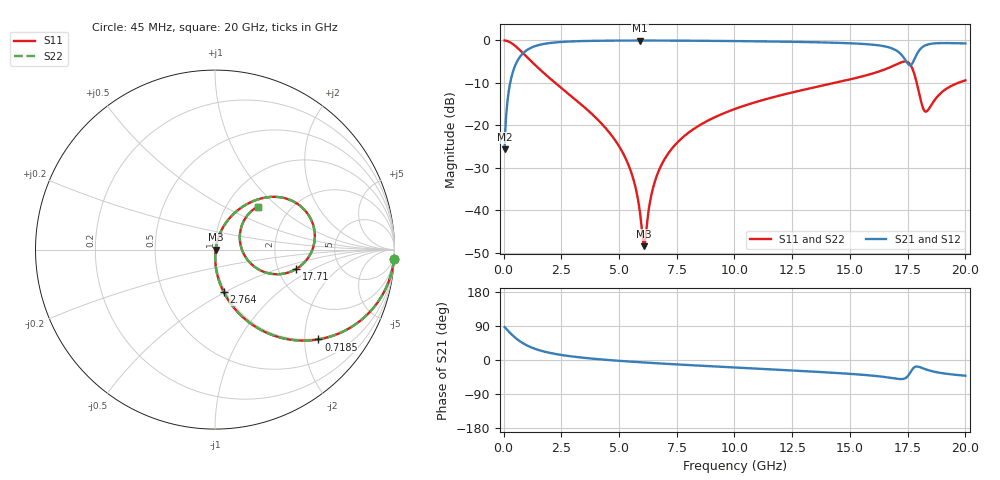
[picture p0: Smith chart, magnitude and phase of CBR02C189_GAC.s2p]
! S-parameter model data by Modelithics Inc.  support@modelithics.com 813-866-6335  Tampa FL USA
! S-Parameter data specifications:
! Substrate: 20-mil Rogers 4350B, substrate thickness, H=0.508mm, Dielectric constant, Er=3.75
! PCB Mounting Pad Footprint: Pad width, PadW=0.32mm , Pad length, PadL=0.37mm , Pad gap, PadG (edge-to-edge)=0.19mm , Reference planes=0.93mm apart
#  GHz  S  MA  R 50
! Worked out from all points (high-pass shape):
!   801 points, 45 MHz to 20 GHz, reference 50 ohm
!   highest |S21| = -0.03 dB at 5.907 GHz (marker M1); lowest = -25.7 dB at 45 MHz (marker M2)
!   |S21| within 3 dB of the highest: 842.1 MHz to 17.17 GHz (16.33 GHz wide, 181 % of centre); 17.92 GHz to end of sweep
!   lowest |S11| = -48.5 dB at 6.081 GHz (marker M3), VSWR 1.01, Z = 50.4 - j0.0664 ohm
!   |S11| at or under -10 dB: 2.238 GHz to 14.34 GHz (12.11 GHz wide, 146 % of centre); 17.89 GHz to 19.69 GHz (1.794 GHz wide, 9.55 % of centre)
!   |S22| runs from -48.5 to 0.0 dB; largest |S21 - S12| = 0
!   S11 on the Smith chart (normalised r, x): 45 MHz: 1, -38; 718.5 MHz: 0.97, -2.33; 2.764 GHz: 0.98, -0.49; 17.71 GHz: 2.52, -0.69; 20 GHz: 1.39, +0.75
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0.045  0.9986 -3.0  0.05217 87.0  0.05217 87.0  0.9986 -3.0
0.294438  0.9459 -19.2  0.3241 70.8  0.3241 70.8  0.9459 -19.2
0.718481  0.7631 -41.0  0.6453 49.0  0.6453 49.0  0.7631 -41.0
1.516681  0.47 -63.4  0.8809 26.4  0.8809 26.4  0.47 -63.4
2.763869  0.2408 -78.5  0.9681 10.9  0.9681 10.9  0.2408 -78.5
3.387462  0.1738 -82.8  0.982 6.3  0.982 6.3  0.1738 -82.8
5.158469  0.04782 -88.7  0.9953 -2.9  0.9953 -2.9  0.04782 -88.7
5.6324  0.02265 -85.6  0.996 -4.8  0.996 -4.8  0.02265 -85.6
5.906781  0.00941 -72.7  0.9961 -5.9  0.9961 -5.9  0.00941 -72.7
6.081387  0.003775 -10.1  0.9961 -6.6  0.9961 -6.6  0.003775 -10.1
6.405656  0.01535 67.6  0.9959 -7.8  0.9959 -7.8  0.01535 67.6
6.704981  0.02849 73.1  0.9955 -8.9  0.9955 -8.9  0.02849 73.1
7.877338  0.07675 73.8  0.9925 -12.9  0.9925 -12.9  0.07675 73.8
10.0225  0.156 68.3  0.9823 -19.8  0.9823 -19.8  0.156 68.3
13.36496  0.2762 57.9  0.9532 -30.5  0.9532 -30.5  0.2762 57.9
16.68248  0.4754 37.5  0.8291 -46.3  0.8291 -46.3  0.4754 37.5
17.40585  0.5642 11.2  0.5843 -47.8  0.5843 -47.8  0.5642 11.2
17.70518  0.4653 -13.4  0.5387 -24.2  0.5387 -24.2  0.4653 -13.4
18.0045  0.2341 -23.1  0.7662 -18.4  0.7662 -18.4  0.2341 -23.1
18.27888  0.1448 10.3  0.8774 -24.6  0.8774 -24.6  0.1448 10.3
19.07708  0.2579 46.5  0.9304 -35.5  0.9304 -35.5  0.2579 46.5
20  0.3382 45.2  0.9213 -41.5  0.9213 -41.5  0.3382 45.2
